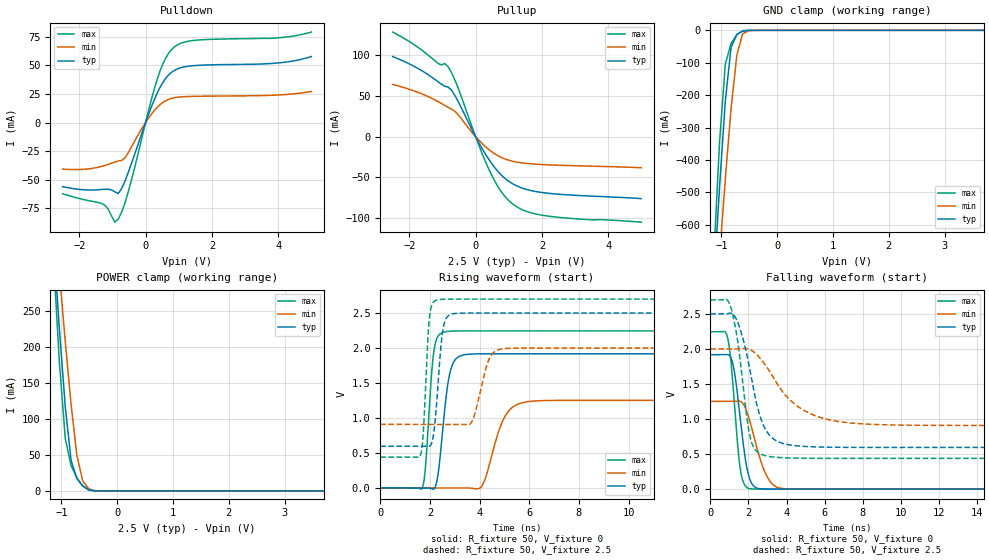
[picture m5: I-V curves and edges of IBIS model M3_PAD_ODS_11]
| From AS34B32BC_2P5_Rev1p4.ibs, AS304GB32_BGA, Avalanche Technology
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[Model] M3_PAD_ODS_11
Model_type I/O
Enable   Active-High
Vinl  =  0.7
Vinh  =  1.8
Vmeas =  1.25
Cref  =  30e-12
| Capacitance   typ   min   max
C_comp   6.259786e-12  5.891456e-12  6.837814e-12
| Variables   typ   min   max
[GND Clamp Reference]   0   0   0
[POWER Clamp Reference]   2.5   2   2.7
[Pulldown Reference]   0   0   0
[Pullup Reference]   2.5   2   2.7
[Temperature Range]   25   125   -40
[Voltage Range]   2.5   2   2.7
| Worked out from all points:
|   slope of the pulldown table from 0 to 0.375 V, typ, clamps not added: 13.9 ohm
|   slope of the pullup table from 0 to 0.375 V, typ, clamps not added: 14.2 ohm
|   GND clamp passes 1 mA (typ) near -0.56 V on its own axis
|   POWER clamp passes 1 mA (typ) near -0.46 V on its own axis
|   falling waveform, R_fixture 50, V_fixture 0: 20-80 % time 523ps typ, 811ps min, 405ps max; typ from 1.92 V to 0 V
|   falling waveform, R_fixture 50, V_fixture 2.5: 20-80 % time 953ps typ, 2.03ns min, 633ps max; typ from 2.5 V to 0.595 V
|   rising waveform, R_fixture 50, V_fixture 0: 20-80 % time 351ps typ, 660ps min, 252ps max; typ from 0 V to 1.92 V
|   rising waveform, R_fixture 50, V_fixture 2.5: 20-80 % time 254ps typ, 460ps min, 186ps max; typ from 0.595 V to 2.5 V
[GND Clamp]
| Voltage   I(typ)   I(min)   I(max)
-2.5V     -5.188A    -4.586A    -6.153A
-1.138V   -783.9mA   -953.3mA   -701.6mA
-1.034V   -484.9mA   -700.5mA   -347mA
-931mV    -219.3mA   -459.7mA   -104.8mA
-827.6mV  -52.73mA   -241.7mA   -40.47mA
-724.1mV  -12.9mA    -76.61mA   -13.47mA
-620.7mV  -2.491mA   -11.2mA    -1.732mA
-517.2mV  -140.5uA   -1.281mA   -29.11uA
-413.8mV  -3.362uA   -98.11uA   -229.5nA
5V        0A         0A         0A
[POWER Clamp]
| Voltage   I(typ)   I(min)   I(max)
-2.5V     2.044A     1.82A      2.427A
-1.138V   339mA      399.6mA    314.6mA
-1.034V   222.7mA    301.1mA    175.8mA
-931mV    116.3mA    206.8mA    72.64mA
-827.6mV  42.71mA    120.3mA    35.15mA
-724.1mV  16.95mA    49.78mA    18.47mA
-620.7mV  7.083mA    14.35mA    7.103mA
-517.2mV  1.86mA     3.351mA    1.319mA
-413.8mV  190.6uA    480.6uA    44.77uA
-310.3mV  6.062uA    46.87uA    467.4nA
5V        0A         0A         0A
[Pulldown]
| Voltage   I(typ)   I(min)   I(max)
-2.5V     -55.99mA   -40.65mA   -62.12mA
-1.345V   -58.47mA   -38.45mA   -70.46mA
-1.138V   -58.16mA   -36.63mA   -75.08mA
-931mV    -60.43mA   -34.49mA   -86.96mA
-827.6mV  -61.95mA   -33.61mA   -84.4mA
-517.2mV  -43.17mA   -26.04mA   -59.93mA
344.8mV   25.28mA    13.14mA    37.23mA
603.4mV   38.43mA    19.08mA    56.07mA
948.3mV   46.68mA    21.99mA    67.55mA
1.638V    49.99mA    22.96mA    72.11mA
3.99V     51.98mA    24.03mA    73.9mA
5V        57.62mA    27.08mA    78.94mA
[Pullup]
| Voltage   I(typ)   I(min)   I(max)
-2.5V     98.48mA    64.18mA    128.6mA
-1.759V   84.36mA    54.81mA    110.5mA
-1.138V   67.71mA    43.27mA    90.34mA
-827.6mV  61.02mA    35.96mA    86.03mA
-517.2mV  42.65mA    26.62mA    58.92mA
86.21mV   -6.586mA   -3.865mA   -9.317mA
431mV     -29.95mA   -16.92mA   -42.83mA
775.9mV   -47.25mA   -25.57mA   -67.74mA
1.121V    -58.06mA   -30.33mA   -82.9mA
1.552V    -65.2mA    -33.03mA   -92.22mA
2.155V    -69.51mA   -34.62mA   -97.61mA
5V        -76.28mA   -38.29mA   -105.3mA
[Ramp]
dV/dt_r   1.1507/0.351025n  0.751452/0.660166n  1.3472/0.251967n
dV/dt_f   1.14297/0.952754n  0.654868/2.03372n  1.35646/0.633338n
R_load = 50
[Falling Waveform]
R_fixture = 50
V_fixture = 0
V_fixture_min = 0
V_fixture_max = 0
| Time   V(typ)   V(min)   V(max)
0s        1.918V     1.252V     2.245V
912ps     1.921V     1.253V     2.157V
1.052ns   1.89V      1.253V     1.906V
1.226ns   1.734V     1.253V     1.361V
1.574ns   1.005V     1.253V     284.2mV
2.007ns   200.2mV    1.032V     10.15mV
2.302ns   36.12mV    737.4mV    2.205mV
2.873ns   2.033mV    237.2mV    497.4uV
3.593ns   476.3uV    18.91mV    392.7uV
21.88ns   1.455uV    104.9nV    -2.134uV
[Falling Waveform]
R_fixture = 50
V_fixture = 2.5
V_fixture_min = 2
V_fixture_max = 2.7
| Time   V(typ)   V(min)   V(max)
0s        2.5V       2V         2.7V
843.4ps   2.501V     2V         2.71V
1.074ns   2.511V     2.001V     2.597V
1.461ns   2.366V     2.001V     2.066V
2.068ns   1.713V     1.995V     772.2mV
2.71ns    964.8mV    1.835V     492.4mV
3.397ns   700.2mV    1.553V     456.1mV
4.41ns    621.8mV    1.216V     443.2mV
6.718ns   597.1mV    965.6mV    439.4mV
21.88ns   595.1mV    908.6mV    439.2mV
[Rising Waveform]
R_fixture = 50
V_fixture = 0
V_fixture_min = 0
V_fixture_max = 0
| Time   V(typ)   V(min)   V(max)
0s        4.27nV     154.6nV    3.596nV
1.696ns   -564.9uV   -264.1uV   3.738mV
2.144ns   -17.68mV   -333.7uV   1.918V
2.54ns    931mV      -395.5uV   2.226V
2.791ns   1.624V     -434.6uV   2.24V
3.067ns   1.853V     -477.6uV   2.244V
4.072ns   1.917V     18.49mV    2.244V
4.951ns   1.917V     975.2mV    2.245V
5.771ns   1.917V     1.222V     2.245V
21.88ns   1.918V     1.252V     2.245V
[Rising Waveform]
R_fixture = 50
V_fixture = 2.5
V_fixture_min = 2
V_fixture_max = 2.7
| Time   V(typ)   V(min)   V(max)
0s        595.1mV    908.6mV    439.2mV
1.619ns   594.5mV    908.1mV    469mV
1.972ns   594.4mV    908mV      2.415V
2.293ns   1.32V      908mV      2.689V
2.54ns    2.296V     907.9mV    2.698V
2.906ns   2.489V     907.8mV    2.699V
3.653ns   2.499V     927.4mV    2.699V
4.365ns   2.499V     1.826V     2.699V
4.913ns   2.499V     1.988V     2.699V
21.88ns   2.5V       2V         2.7V
